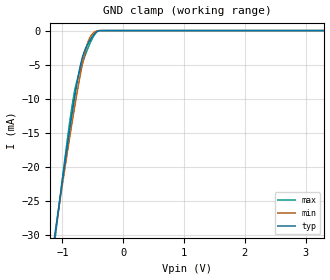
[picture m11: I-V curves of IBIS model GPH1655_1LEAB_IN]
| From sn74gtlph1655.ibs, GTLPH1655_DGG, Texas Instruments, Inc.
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[Model]   GPH1655_1LEAB_IN
Model_type  Input
Vinl=0.69
Vinh=1.05
| variable   typ   min   max
C_comp   3.01pF   2.24pF   3.95pF
[Temperature Range]   40   100   -40
| Ambient temperature   25   85   -40
[Voltage range]   3.3   3.15   3.45
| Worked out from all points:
|   GND clamp passes 1 mA (typ) near -0.52 V on its own axis
[GND Clamp]
| GPH1655_1LEAB_IN
|   Voltage   I(typ)   I(min)   I(max)
-5.5V     -348mA     -320.7mA   -389.8mA
-1.11V    -29.09mA   -29.13mA   -29.74mA
-1.07V    -26.47mA   -26.72mA   -26.78mA
-895mV    -15.37mA   -16.48mA   -14.42mA
-840mV    -12.09mA   -13.41mA   -10.99mA
-800mV    -9.813mA   -11.24mA   -8.913mA
-725mV    -5.999mA   -7.402mA   -6.269mA
-660mV    -3.579mA   -4.448mA   -4.491mA
-575mV    -1.843mA   -1.603mA   -2.457mA
-485mV    -638.7uA   -307.2uA   -791.6uA
-390mV    -8.587uA   -16.56uA   -7.146uA
3.3V      166.6pA    582.8pA    1.325nA
